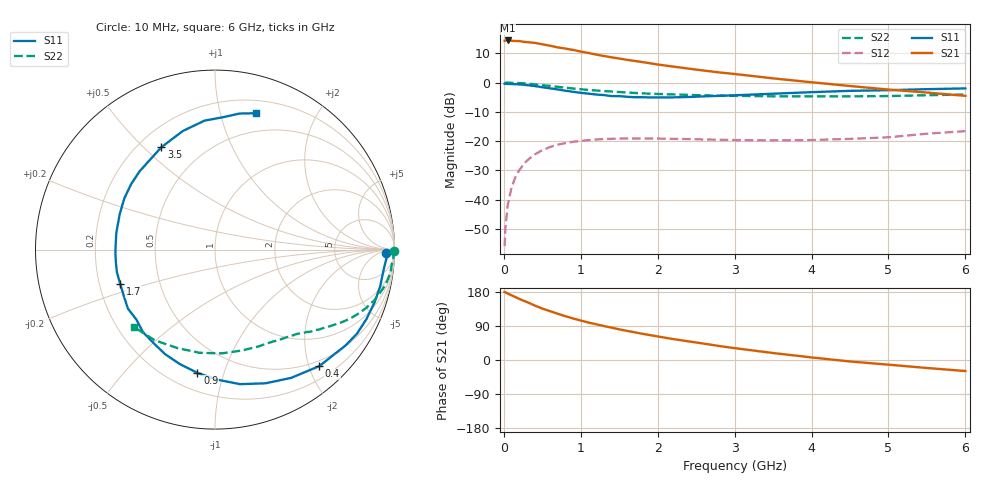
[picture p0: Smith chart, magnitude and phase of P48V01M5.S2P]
! SIEMENS Small Signal Semiconductors
! BFP182
! Si NPN RF Bipolar Junction Transistor in SOT143
! VCE = 8 V  IC = 1.5 mA
! Common Emitter S-Parameters:  March  1996
# GHz  S  MA  R  50
!  f  S11  S21  S12  S22
! GHz  MAG  ANG  MAG  ANG  MAG  ANG  MAG  ANG
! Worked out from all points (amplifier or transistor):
!   36 points, 10 MHz to 6 GHz, reference 50 ohm
!   highest |S21| = 14.4 dB at 50 MHz (marker M1)
!   |S21| within 3 dB of that: start of sweep to 848.7 MHz
!   unconditionally stable (mu >= 1): 2.446 GHz to end of sweep
!   at 250 MHz: K = 0.11, MSG = 21.1 dB, |S12| = -28.2 dB
!   at 1.4 GHz: K = 0.60, MSG = 13.9 dB, |S12| = -19.2 dB
!   at 6 GHz: K = 1.01, MAG = 5.4 dB, |S12| = -16.6 dB
!   S11 on the Smith chart (normalised r, x): 10 MHz: 34, -15; 400 MHz: 0.40, -2.17; 900 MHz: 0.31, -0.82; 1.7 GHz: 0.29, -0.16; 3.5 GHz: 0.29, +0.57; 6 GHz: 0.32, +1.30
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0.01  0.9518 -1.2  5.17 179.3  0.0016 83.4  0.9967 -0.4
0.02  0.9578 -2.5  5.198 178.7  0.0032 88.7  0.9901 -0.9
0.05  0.9475 -6.1  5.233 175.4  0.008 88.7  0.9954 -2.4
0.1  0.9428 -12.5  5.158 170.7  0.016 82.1  0.9882 -4.7
0.15  0.9363 -18.5  5.117 166.2  0.0241 78.0  0.9864 -7.0
0.2  0.9282 -24.7  5.115 161.4  0.0317 75.5  0.9789 -9.4
0.4  0.8712 -48.2  4.764 143.9  0.0589 61.6  0.9315 -17.6
0.5  0.8312 -59.3  4.504 135.8  0.0698 55.2  0.9013 -21.3
0.6  0.7963 -69.3  4.256 128.9  0.0789 50.0  0.8727 -24.3
0.7  0.7624 -79.5  3.986 122.1  0.0868 45.0  0.8448 -27.1
0.8  0.725 -88.9  3.803 115.6  0.0922 40.4  0.8162 -29.6
0.9  0.6938 -98.1  3.604 109.6  0.0973 36.4  0.7899 -31.8
1.1  0.6454 -115.5  3.202 98.9  0.1038 29.8  0.7472 -35.7
1.4  0.5863 -138.4  2.694 85.3  0.1093 21.7  0.7025 -40.6
1.7  0.5615 -160.1  2.339 73.1  0.1103 16.3  0.6626 -44.9
1.9  0.5568 -172.6  2.134 65.7  0.1103 13.4  0.6454 -47.8
2.2  0.5578 170.3  1.873 55.3  0.109 10.5  0.6258 -52.1
2.8  0.5925 142.2  1.489 36.9  0.1053 7.6  0.5962 -61.8
3.5  0.6438 117.7  1.178 18.4  0.1027 8.2  0.5816 -75.3
4.5  0.721 94.6  0.872 -3.9  0.109 12.9  0.5813 -98.6
5.5  0.7702 79.8  0.674 -21.1  0.1336 16.9  0.6069 -123.8
6  0.7937 73.2  0.592 -29.1  0.1476 14.8  0.6243 -136.4
